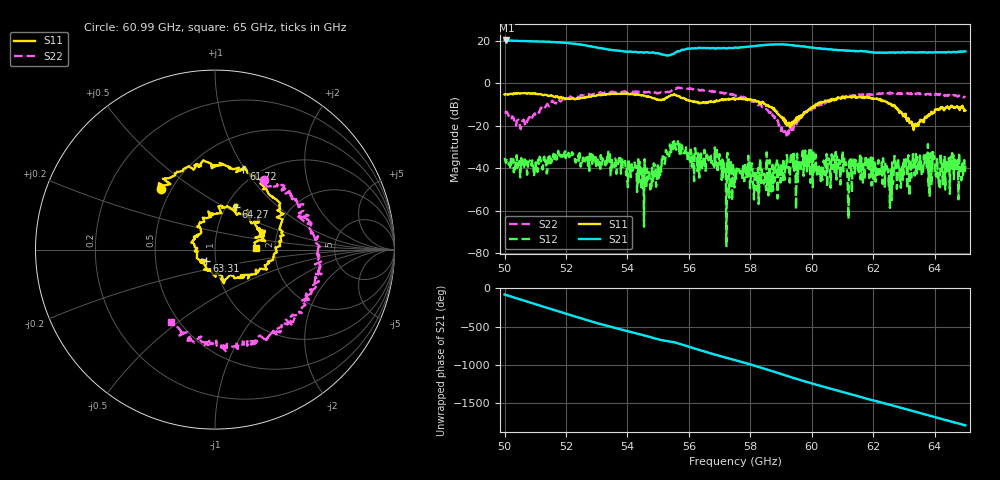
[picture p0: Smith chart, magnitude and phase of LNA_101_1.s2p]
! Created Tue Jul 15 12:28:44 2008
# hz S ma R 50
! 2 Port Network Data from blockName block
! freq  magS11  angS11  magS21  angS21  magS12  angS12  magS22  angS22
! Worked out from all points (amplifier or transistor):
!   801 points, 50 GHz to 65 GHz, reference 50 ohm
!   highest |S21| = 20.3 dB at 50.06 GHz (marker M1)
!   |S21| within 3 dB of that: start of sweep to 52.87 GHz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
!   unconditionally stable (mu >= 1): start of sweep to 55.44 GHz; 55.79956 GHz to 55.89539 GHz; 55.91 GHz to end of sweep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
!   at 52.49 GHz: K = 3.02, MAG = 20.5 dB, |S12| = -38.1 dB
!   at 57.5 GHz: K = 6.98, MAG = 19.3 dB, |S12| = -44.5 dB
!   at 65 GHz: K = 5.92, MAG = 16.4 dB, |S12| = -39.0 dB
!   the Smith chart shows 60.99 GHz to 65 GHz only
!   S11 on the Smith chart (normalised r, x): 60.99 GHz: 0.44, +0.38; 61.72 GHz: 0.85, +0.99; 63.31 GHz: 0.90, -0.11; 64.27 GHz: 1.11, +0.56; 65 GHz: 1.60, +0.03
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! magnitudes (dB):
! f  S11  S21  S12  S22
! 50 GHz  -5.2  20.3  -35.2  -13.7
! 50.06 GHz  -5.1  20.3  -37.4  -13.6
! 50.58 GHz  -4.7  20.0  -36.3  -17.6
! 52.51 GHz  -6.9  18.3  -36.2  -5.6
! 54.22 GHz  -5.2  14.9  -37.5  -4.0
! 54.54 GHz  -5.7  14.4  -67.6  -4.1
! 55.01 GHz  -7.7  14.3  -44.8  -4.7
! 55.51 GHz  -5.1  14.1  -27.3  -2.9
! 56.36 GHz  -9.4  16.7  -34.4  -3.1
! 56.92 GHz  -8.3  16.6  -38.1  -4.1
! 57.14 GHz  -7.6  16.8  -42.4  -4.9
! 57.5 GHz  -7.2  16.9  -44.5  -5.8
! 58.62 GHz  -10.9  18.3  -36.2  -13.7
! 59.15 GHz  -17.4  18.3  -39.0  -22.8
! 60.01 GHz  -11.5  16.9  -39.2  -12.0
! 60.99 GHz  -6.9  15.7  -37.0  -6.5
! 61.23 GHz  -6.4  15.4  -35.6  -6.3
! 61.72 GHz  -6.4  15.1  -45.6  -5.4
! 62.51 GHz  -9.2  14.6  -48.3  -4.6
! 63.31 GHz  -22.1  14.6  -37.6  -4.8
! 64.27 GHz  -11.6  14.7  -47.7  -5.3
! 65 GHz  -12.8  15.1  -39.0  -6.5
